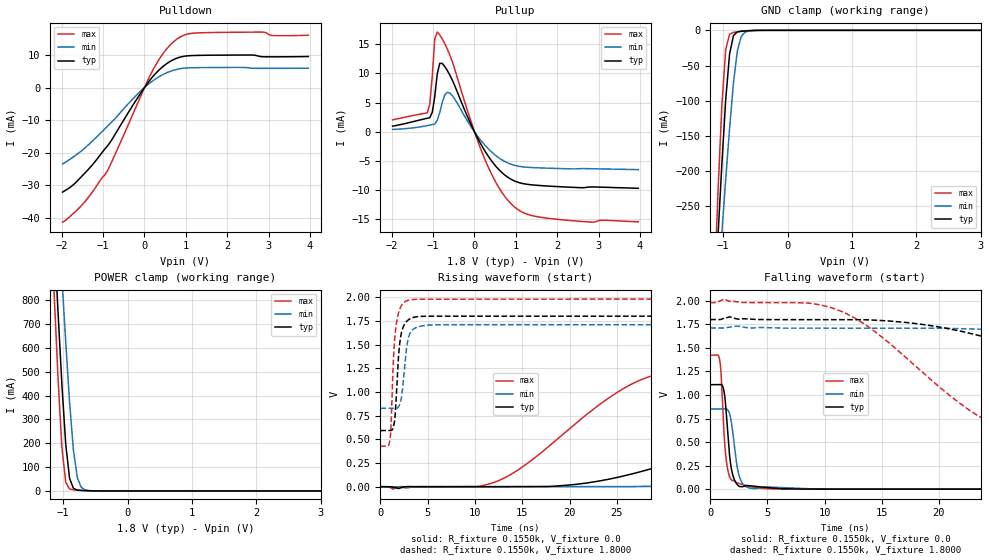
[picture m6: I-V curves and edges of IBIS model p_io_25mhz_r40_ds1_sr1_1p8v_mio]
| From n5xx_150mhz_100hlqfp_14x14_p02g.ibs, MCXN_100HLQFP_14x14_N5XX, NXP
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[Model] p_io_25mhz_r40_ds1_sr1_1p8v_mio
|   Model p_io_25mhz_r40_ds1_sr1_1p8v_mio
| This model was characterised for following simulation conditions:
| External (pad) voltage:
|   - Typ: 1.8V,   - Min: 1.71V,   - Max: 1.98V
| Library cells for typ/min/max conditions are connected as defined below:
|  pad - External Pad
|  ipp_do_lv - Core Input
|  ipp_obe_lv - Output Buffer Enable
|  IOGC - NC
|  REFH3V3 - REFH3V3
|  REFL3V3 - REFL3V3
|  ZI - NC
|  abut_ncal_vddio[1] - vssio vddio vddio
|  abut_ncal_vddio[2] - vddio vddio vssio
|  abut_ncal_vddio[3] - vddio
|  abut_ncal_vddio[4] - vssio vddio vddio
|  abut_ncal_vddio[5] - vddio vddio vssio
|  abut_ncal_vddio[6] - vddio
|  abut_pcal_vddio[1] - vssio
|  abut_pcal_vddio[2] - vddio vssio vddio
|  abut_pcal_vddio[3] - vssio
|  abut_pcal_vddio[4] - vssio
|  abut_pcal_vddio[5] - vddio vssio vddio
|  abut_pcal_vddio[6] - vssio
|  ipp_do_1p8v - ipp_do_1p8v
|  ipp_dse_lv - vdd_lv
|  ipp_eftd_lv - NC
|  ipp_ina_mux_vddio - NC
|  ipp_ina_mux_vddio[0] - NC
|  ipp_ina_mux_vddio[1] - NC
|  ipp_ina_r0_vddio - NC
|  ipp_ina_r0a_vddio - NC
|  ipp_ina_r0b_vddio - NC
|  ipp_ina_r0c_vddio - NC
|  ipp_ina_r0d_vddio - NC
|  ipp_ina_r0e_vddio - NC
|  ipp_ina_r0f_vddio - NC
|  ipp_ina_r300_vddio - NC
|  ipp_ina_r300a_vddio - NC
|  ipp_ina_r300b_vddio - NC
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Model_type I/O
Polarity   Non-Inverting
Enable   Active-High
Vinl =   0.5400V
Vinh =   1.2600V
Vmeas =  0.9000V
Cref =   30.0000pF
Rref =   1.0000M
Vref =   1.8000V
C_comp   1.7117pF   1.6504pF   1.7864pF
|C_comp_pullup   0.6276pF   0.6567pF   0.6008pF
|C_comp_pulldown   0.8230pF   0.8663pF   0.7899pF
[Model Spec]
| variable   typ   min   max
Vinh   1.2600V   1.1970V   1.3860V
Vinl   0.5400V   0.5130V   0.5940V
[Temperature Range]   25.0000   0.1250k   -40.0000
[Voltage Range]   1.8000V   1.7100V   1.9800V
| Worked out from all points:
|   slope of the pulldown table from 0 to 0.27 V, typ, clamps not added: 62.5 ohm
|   slope of the pullup table from 0 to 0.27 V, typ, clamps not added: 77.5 ohm
|   GND clamp passes 1 mA (typ) near -0.68 V on its own axis
|   POWER clamp passes 1 mA (typ) near -0.63 V on its own axis
|   rising waveform, R_fixture 0.1550k, V_fixture 0.0: 20-80 % time 23.2ns typ, 43.7ns min, 11.7ns max; typ from 0 V to 1.11 V
|   rising waveform, R_fixture 0.1550k, V_fixture 1.8000: 20-80 % time 491ps typ, 569ps min, 460ps max; typ from 0.592 V to 1.8 V
|   falling waveform, R_fixture 0.1550k, V_fixture 0.0: 20-80 % time 493ps typ, 583ps min, 440ps max; typ from 1.11 V to 0 V
|   falling waveform, R_fixture 0.1550k, V_fixture 1.8000: 20-80 % time 19.3ns typ, 37.6ns min, 9.61ns max; typ from 1.8 V to 0.592 V
[Pulldown]
|Voltage   I(typ)   I(min)   I(max)
-1.98V    -32.06mA   -23.44mA   -41.28mA
-1.5V     -27mA      -19.16mA   -35.86mA
-900mV    -17.97mA   -11.92mA   -25.7mA
-180mV    -3.435mA   -2.171mA   -5.239mA
180mV     3.035mA    1.877mA    4.805mA
480mV     6.794mA    4.206mA    10.94mA
780mV     8.992mA    5.567mA    14.82mA
1.02V     9.698mA    6.006mA    16.34mA
1.38V     9.876mA    6.116mA    16.79mA
2.88V     9.432mA    5.88mA     16.99mA
3.12V     9.425mA    5.883mA    15.91mA
3.96V     9.519mA    5.936mA    16.03mA
[Pullup]
|Voltage   I(typ)   I(min)   I(max)
-1.98V    967.3uA    399.6uA    2.046mA
-1.14V    2.322mA    1.064mA    3.245mA
-1.08V    2.417mA    1.15mA     4.767mA
-1.02V    3.36mA     1.241mA    9.562mA
-960mV    6.043mA    1.333mA    15.9mA
-900mV    9.924mA    1.975mA    17.07mA
-780mV    11.72mA    5.036mA    15.9mA
-600mV    9.761mA    6.668mA    13.21mA
240mV     -3.146mA   -2.19mA    -4.535mA
900mV     -8.187mA   -5.593mA   -12.43mA
1.68V     -9.242mA   -6.203mA   -14.71mA
3.96V     -9.671mA   -6.472mA   -15.42mA
[GND_clamp]
|Voltage   I(typ)   I(min)   I(max)
-1.98V    -2.014A    -1.664A    -2.513A
-1.14V    -398mA     -446.7mA   -367.4mA
-1.08V    -291.8mA   -366.3mA   -229.6mA
-1.02V    -190.1mA   -287.6mA   -106.6mA
-960mV    -98.09mA   -211.4mA   -27.19mA
-900mV    -33.41mA   -139.1mA   -5.497mA
-840mV    -7.43mA    -74.57mA   -2.952mA
-780mV    -2.331mA   -29.72mA   -2.122mA
-720mV    -1.309mA   -8.82mA    -1.477mA
-660mV    -833.8uA   -2.501mA   -940.4uA
-360mV    -6.03uA    -22.55uA   -2.113uA
3.96V     0A         0A         0A
[POWER_clamp]
|Voltage   I(typ)   I(min)   I(max)
-1.98V    5.618A     5.349A     6.084A
-1.14V    1.071A     1.443A     829.6mA
-1.08V    754.2mA    1.168A     476.4mA
-1.02V    449mA      895.6mA    184.6mA
-960mV    195.8mA    625.5mA    36.79mA
-900mV    52.44mA    371.1mA    7.808mA
-840mV    10.74mA    170.2mA    4.435mA
-780mV    3.619mA    56.22mA    3.182mA
-720mV    2.074mA    15.04mA    2.195mA
-660mV    1.306mA    4.299mA    1.376mA
-360mV    5.079uA    27.62uA    1.341uA
3.96V     0A         0A         0A
[Ramp]
| variable   typ   min   max
dV/dt_r  0.6653/23.1910n   0.5082/43.7382n   0.8533/11.7359n
dV/dt_f  0.7247/19.3068n   0.5284/37.5906n   0.9319/9.6107n
R_load = 0.1550k
[Rising Waveform]
R_fixture= 0.1550k
V_fixture= 0.0
V_fixture_min= 0.0
V_fixture_max= 0.0
|time   V(typ)   V(min)   V(max)
0s        440.4pV    137.8nV    11.97pV
11.75ns   -27.95uV   -9.347uV   36.03mV
20.55ns   23.01mV    67.92uV    658.3mV
27.53ns   159mV      2.472mV    1.128V
41.09ns   596.6mV    73.34mV    1.346V
50.89ns   854mV      181.2mV    1.386V
60.55ns   968.5mV    311.8mV    1.404V
81.7ns    1.059V     585.5mV    1.418V
103.2ns   1.09V      723.9mV    1.421V
235ns     1.109V     847mV      1.422V
[Rising Waveform]
R_fixture= 0.1550k
V_fixture= 1.8000
V_fixture_min= 1.7100
V_fixture_max= 1.9800
|time   V(typ)   V(min)   V(max)
0s        592.1mV    827.1mV    426.8mV
1.033ns   591.9mV    827.2mV    500.8mV
1.138ns   592.2mV    827.2mV    644.6mV
1.454ns   660.8mV    827.1mV    1.458V
1.603ns   800.1mV    826.8mV    1.643V
1.865ns   1.284V     835.3mV    1.81V
2.347ns   1.665V     1.027V     1.928V
2.848ns   1.751V     1.511V     1.964V
3.501ns   1.786V     1.663V     1.976V
235ns     1.8V       1.71V      1.98V
[Falling Waveform]
R_fixture= 0.1550k
V_fixture= 0.0
V_fixture_min= 0.0
V_fixture_max= 0.0
|time   V(typ)   V(min)   V(max)
0s        1.109V     850.8mV    1.422V
829.3ps   1.11V      850.8mV    1.367V
949ps     1.111V     850.8mV    1.216V
1.304ns   944.2mV    853.5mV    421.1mV
1.701ns   343.3mV    794.7mV    127.8mV
2.072ns   110.8mV    495.9mV    87.26mV
2.381ns   45.69mV    219mV      66.28mV
2.7ns     26.29mV    85.72mV    52.76mV
4.981ns   16.6mV     23.67mV    5.194mV
235ns     99nV       1.877uV    16.18nV
[Falling Waveform]
R_fixture= 0.1550k
V_fixture= 1.8000
V_fixture_min= 1.7100
V_fixture_max= 1.9800
|time   V(typ)   V(min)   V(max)
0s        1.8V       1.71V      1.98V
10.81ns   1.8V       1.71V      1.918V
14.29ns   1.795V     1.71V      1.683V
24.11ns   1.612V     1.696V     733.2mV
35.6ns    1.147V     1.605V     504.8mV
42.78ns   883.4mV    1.51V      470.2mV
51.12ns   749.3mV    1.374V     450.5mV
68.67ns   653.7mV    1.095V     434.2mV
90.34ns   615.5mV    945.8mV    428.7mV
235ns     592.2mV    829.4mV    426.8mV
